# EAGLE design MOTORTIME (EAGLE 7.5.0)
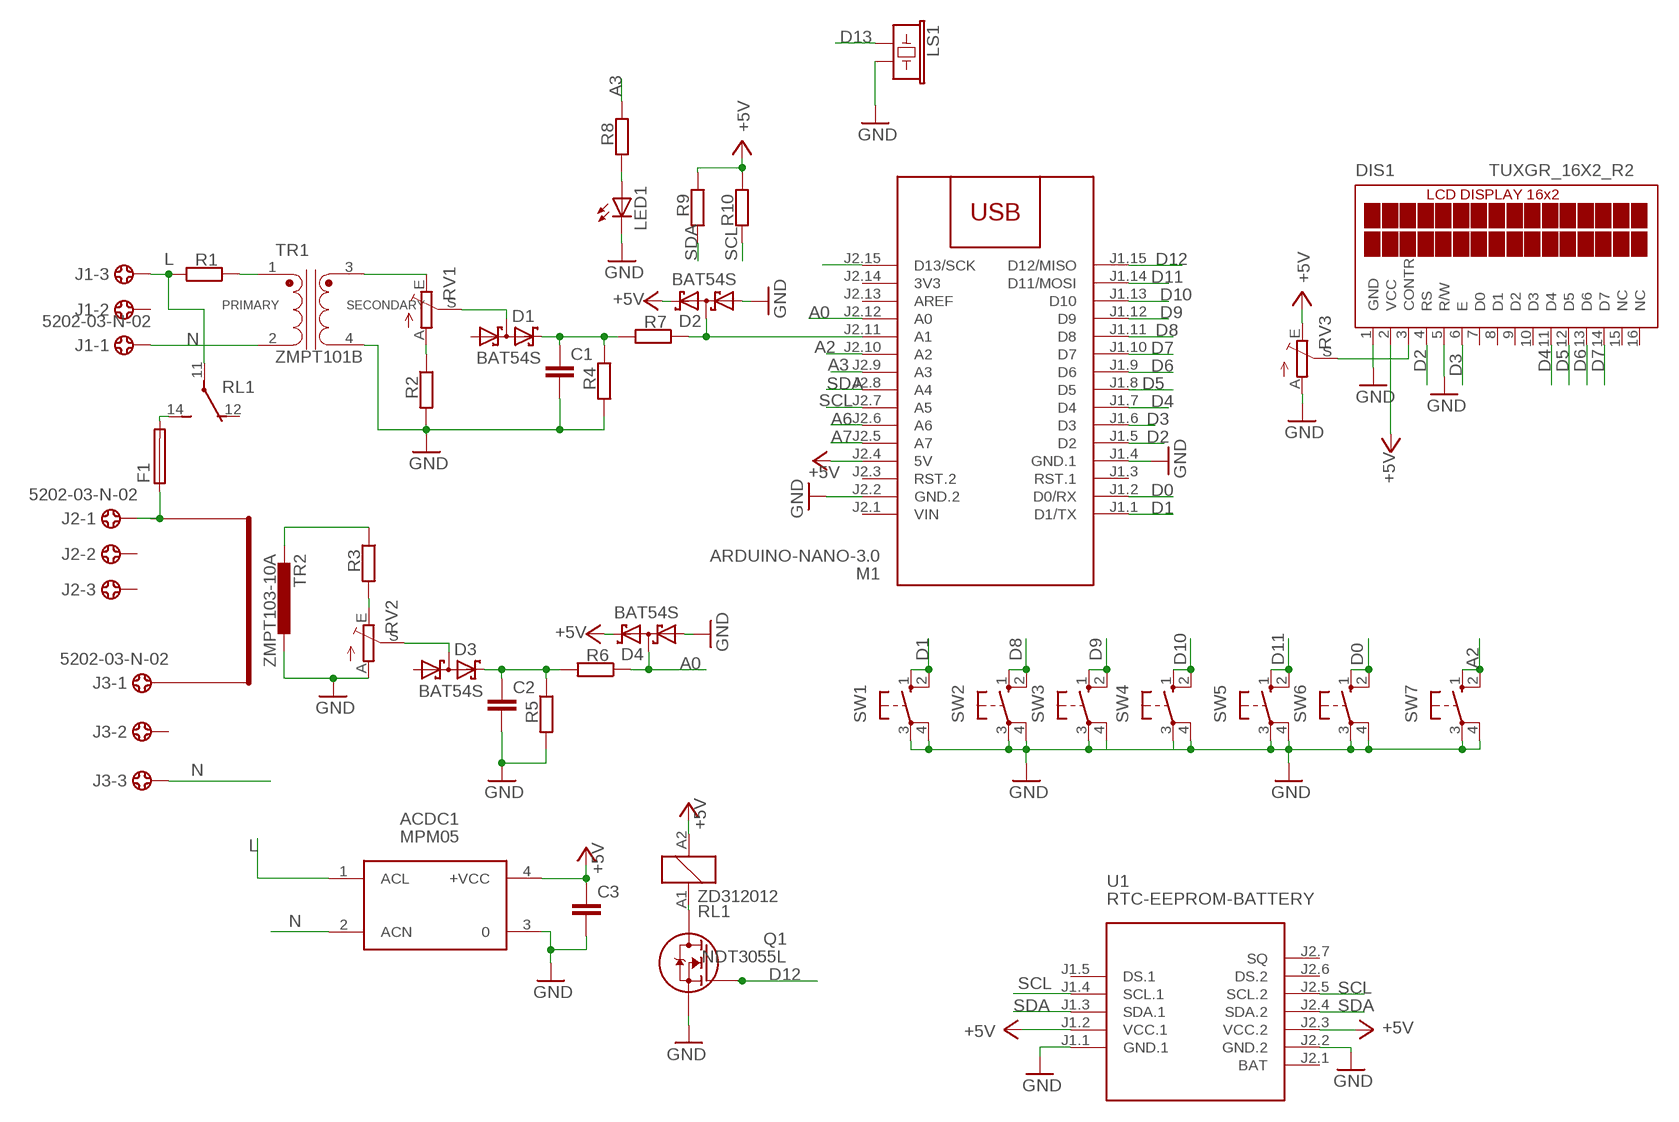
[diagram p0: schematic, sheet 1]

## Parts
ACDC1  MPM05  [MPM05]
C1  C-EUC1206  [C1206]
C2  C-EUC1206  [C1206]
C3  C-EUC1206  [C1206]
D1  BAT54S  [SOT23]
D2  BAT54S  [SOT23]
D3  BAT54S  [SOT23]
D4  BAT54S  [SOT23]
DIS1  TUXGR_16X2_R2  [TUXGR_16X2_R2]
F1  SH22,5A  [SH22,5A]
J1  5202-03-N-02  [5202-03-N-02]
J2  5202-03-N-02  [5202-03-N-02]
J3  5202-03-N-02  [5202-03-N-02]
LED1  LED5MM  [LED5MM]
LS1  BUZZER-PTH_NO_SILK  [BUZZER-12MM-NS]
M1  ARDUINO-NANO-3.0  [ARDUINO-NANO-3.0]
Q1  NDT3055L  [SOT223-4]
R1  R-EU_R1206  [R1206]
R2  R-EU_R1206  [R1206]
R3  R-EU_R1206  [R1206]
R4  R-EU_R1206  [R1206]
R5  R-EU_R1206  [R1206]
R6  R-EU_R1206  [R1206]
R7  R-EU_R1206  [R1206]
R8  R-EU_R1206  [R1206]
R9  R-EU_R1206  [R1206]
R10  R-EU_R1206  [R1206]
RL1  ZD312012  [ZD1]
RV1  TRIM_EU-B64W  [B64W]
RV2  TRIM_EU-B64W  [B64W]
RV3  TRIM_EU-B64W  [B64W]
SW1  10-XX  [B3F-10XX]
SW2  10-XX  [B3F-10XX]
SW3  10-XX  [B3F-10XX]
SW4  10-XX  [B3F-10XX]
SW5  10-XX  [B3F-10XX]
SW6  10-XX  [B3F-10XX]
SW7  10-XX  [B3F-10XX]
TR1  ZMPT101B  [XFMR_ZMPT101B]
TR2  ZMPT103-10A  [ZMPT103-10A]
U1  RTC-EEPROM-BATTERY  [RTC-EEPROM-BATTERY]

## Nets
+5V: ACDC1.4(+VCC) C3.1 D2.2(C2) D4.2(C2) DIS1.2(VCC) M1.J2.4(5V) R9.1 R10.1 RL1.A2 RV3.E U1.J1.2(VCC.1) U1.J2.3(VCC.2)
A0: D4.3(C1A2) M1.J2.12(A0) R6.1
A2: M1.J2.10(A2) SW7.1(S) SW7.2(S1)
A3: M1.J2.9(A3) R8.1
A6: M1.J2.6(A6)
A7: M1.J2.5(A7)
D0: M1.J1.2(D0/RX) SW6.1(S) SW6.2(S1)
D1: M1.J1.1(D1/TX) SW1.1(S) SW1.2(S1)
D2: DIS1.4(RS) M1.J1.5(D2)
D3: DIS1.6(E) M1.J1.6(D3)
D4: DIS1.11(D4) M1.J1.7(D4)
D5: DIS1.12(D5) M1.J1.8(D5)
D6: DIS1.13(D6) M1.J1.9(D6)
D7: DIS1.14(D7) M1.J1.10(D7)
D8: M1.J1.11(D8) SW2.1(S) SW2.2(S1)
D9: M1.J1.12(D9) SW3.1(S) SW3.2(S1)
D10: M1.J1.13(D10) SW4.1(S) SW4.2(S1)
D11: M1.J1.14(D11/MOSI) SW5.1(S) SW5.2(S1)
D12: M1.J1.15(D12/MISO) Q1.1(G)
D13: LS1.+ M1.J2.15(D13/SCK)
GND: ACDC1.3 C1.2 C2.2 C3.2 D2.1(A1) D4.1(A1) DIS1.1(GND) DIS1.5(R/W) LED1.K(C) LS1.- M1.J1.4(GND.1) M1.J2.2(GND.2) Q1.3(S) R2.2 R4.2 R5.2 RV2.A RV3.A SW1.3(P) SW1.4(P1) SW2.3(P) SW2.4(P1) SW3.3(P) SW3.4(P1) SW4.3(P) SW4.4(P1) SW5.3(P) SW5.4(P1) SW6.3(P) SW6.4(P1) SW7.3(P) SW7.4(P1) TR1.4 TR2.P$2 U1.J1.1(GND.1) U1.J2.2(GND.2)
L: ACDC1.1(ACL) J1.3 R1.2 RL1.11(2:P)
N: ACDC1.2(ACN) J1.1 J3.3 TR1.2
N$1: R2.1 RV1.A
N$2: R3.1 TR2.P$1
N$3: R3.2 RV2.E
N$4: F1.2 RL1.14(2:S)
N$5: R1.1 TR1.1
N$6: RV1.E TR1.3
N$7: C1.1 D1.2(C2) R4.1 R7.2
N$8: D1.3(C1A2) RV1.S
N$9: D2.3(C1A2) M1.J2.11(A1) R7.1
N$10: F1.1 J2.1
N$11: D3.3(C1A2) RV2.S
N$12: Q1.2(D) Q1.4(D) RL1.A1
N$13: C2.1 D3.2(C2) R5.1 R6.2
N$14: DIS1.3(CONTR) RV3.S
N$15: LED1.A R8.2
SCL: M1.J2.7(A5) R10.2 U1.J1.4(SCL.1) U1.J2.5(SCL.2)
SDA: M1.J2.8(A4) R9.2 U1.J1.3(SDA.1) U1.J2.4(SDA.2)
Unconnected: D1.1(A1) D3.1(A1) DIS1.7(D0) DIS1.8(D1) DIS1.9(D2) DIS1.10(D3) DIS1.15(NC) DIS1.16(NC) J1.2 J2.2 J2.3 J3.1 J3.2 M1.J1.3(RST.1) M1.J2.3(RST.2) M1.J2.13(AREF) RL1.12(2:O) U1.J1.5(DS.1) U1.J2.1(BAT) U1.J2.6(DS.2) U1.J2.7(SQ)

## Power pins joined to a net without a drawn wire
3V3: M1.J2.14(3V3)
VIN: M1.J2.1(VIN)

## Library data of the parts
ACDC1 = acdc:MPM05: AC DC Converter 5W
C1-C3 = rcl:C-EU: CAPACITOR, European symbol
D1-D4 = diode:BAT54S: Schottky Diodes Pin connection corrected 2011-05-04 Source: Fairchild .. BAT54.pdf
DIS1 = display-lcd:TUXGR_16X2_R2: Tuxgraphics LCD display 16x2 characters reflective, without background light Source: tuxgr_12x2_r2.pdf; OC_FARNELL: unknown; OC_NEWARK: unknown
F1 = fuse:SH22,5A: FUSE HOLDER; MPN: 0031.7701.11; OC_FARNELL: unknown; OC_NEWARK: 04F1224
J1-J3 = con-ebyelectro:5202-03-N-02: Barrier Blocks Sreies 5202 Source: http://www.ebyelectro.com/PDF/5202-XX-N-02.pdf; OC_FARNELL: unknown; OC_NEWARK: unknown
LED1 = led:LED: LED
LS1 = SparkFun-Electromechanical:BUZZER: Buzzer; PROD_ID: COMP-08253; SF_SKU: COM-07950
M1 = diy-modules:ARDUINO-NANO-3.0: Arduino Nano 3.0 and compatible devices More details available here: https://www.arduino.cc/en/Main/ArduinoBoardNano Click here to find device on ebay.com
Q1 = NDT3055L:NDT3055L: Trans MOSFET N-CH 60V 4A 4-Pin(3+Tab) SOT-223 Trans MOSFET N-CH 60V 4A 4-Pin(3+Tab) SOT-223 Check availability; AVAILABILITY: In Stock; CHECK_PRICES: https://www.snapeda.com/parts/NDT3055L/Onsemi/view-part/?ref=eda; DESCRIPTION: Trans MOSFET N-CH 60V 4A 4-Pin(3+Tab) SOT-223 Trans MOSFET N-CH 60V 4A 4-Pin(3+Tab) SOT-223; MF: ON; MP: NDT3055L; PACKAGE: SOT-223-4 Fairchild Semiconductor; PRICE: None; SNAPEDA_LINK: https://www.snapeda.com/parts/NDT3055L/Onsemi/view-part/?ref=snap
R1-R10 = rcl:R-EU_: RESISTOR, European symbol
RL1 = relay:ZD?1*: Power Relay SCHRACK 1 pole 30 A Source: http://www.schrack.com/.. 5848.pdf; OC_FARNELL: unknown; OC_NEWARK: unknown
RV1-RV3 = pot:TRIM_EU-: POTENTIOMETER
SW1-SW7 = switch-omron:10-XX: OMRON SWITCH; MPN: B3F-1000; OC_FARNELL: 176432; OC_NEWARK: 36M3542
TR1 = ZMPT101B:ZMPT101B: Check availability; AVAILABILITY: Not in stock; CHECK_PRICES: https://www.snapeda.com/parts/ZMPT101B/Qingxian+Zeming+Langxi+Electronic/view-part/?ref=eda; DESCRIPTION: Current-type Voltage Transformer; MF: Qingxian Zeming Langxi Electronic; MP: ZMPT101B; PACKAGE: None; PRICE: None; SNAPEDA_LINK: https://www.snapeda.com/parts/ZMPT101B/Qingxian+Zeming+Langxi+Electronic/view-part/?ref=snap
TR2 = diy-modules:ZMPT103-10A
U1 = diy-modules:RTC-EEPROM-BATTERY: RTC Module with Battery and EEPROM based on DS1307 and AT24C32 chips More details available here: http://henrysbench.capnfatz.com/henrys-bench/arduino-sensors-and-input/arduino-tiny-rtc-d1307-tutorial/ Click here to find device on ebay.com

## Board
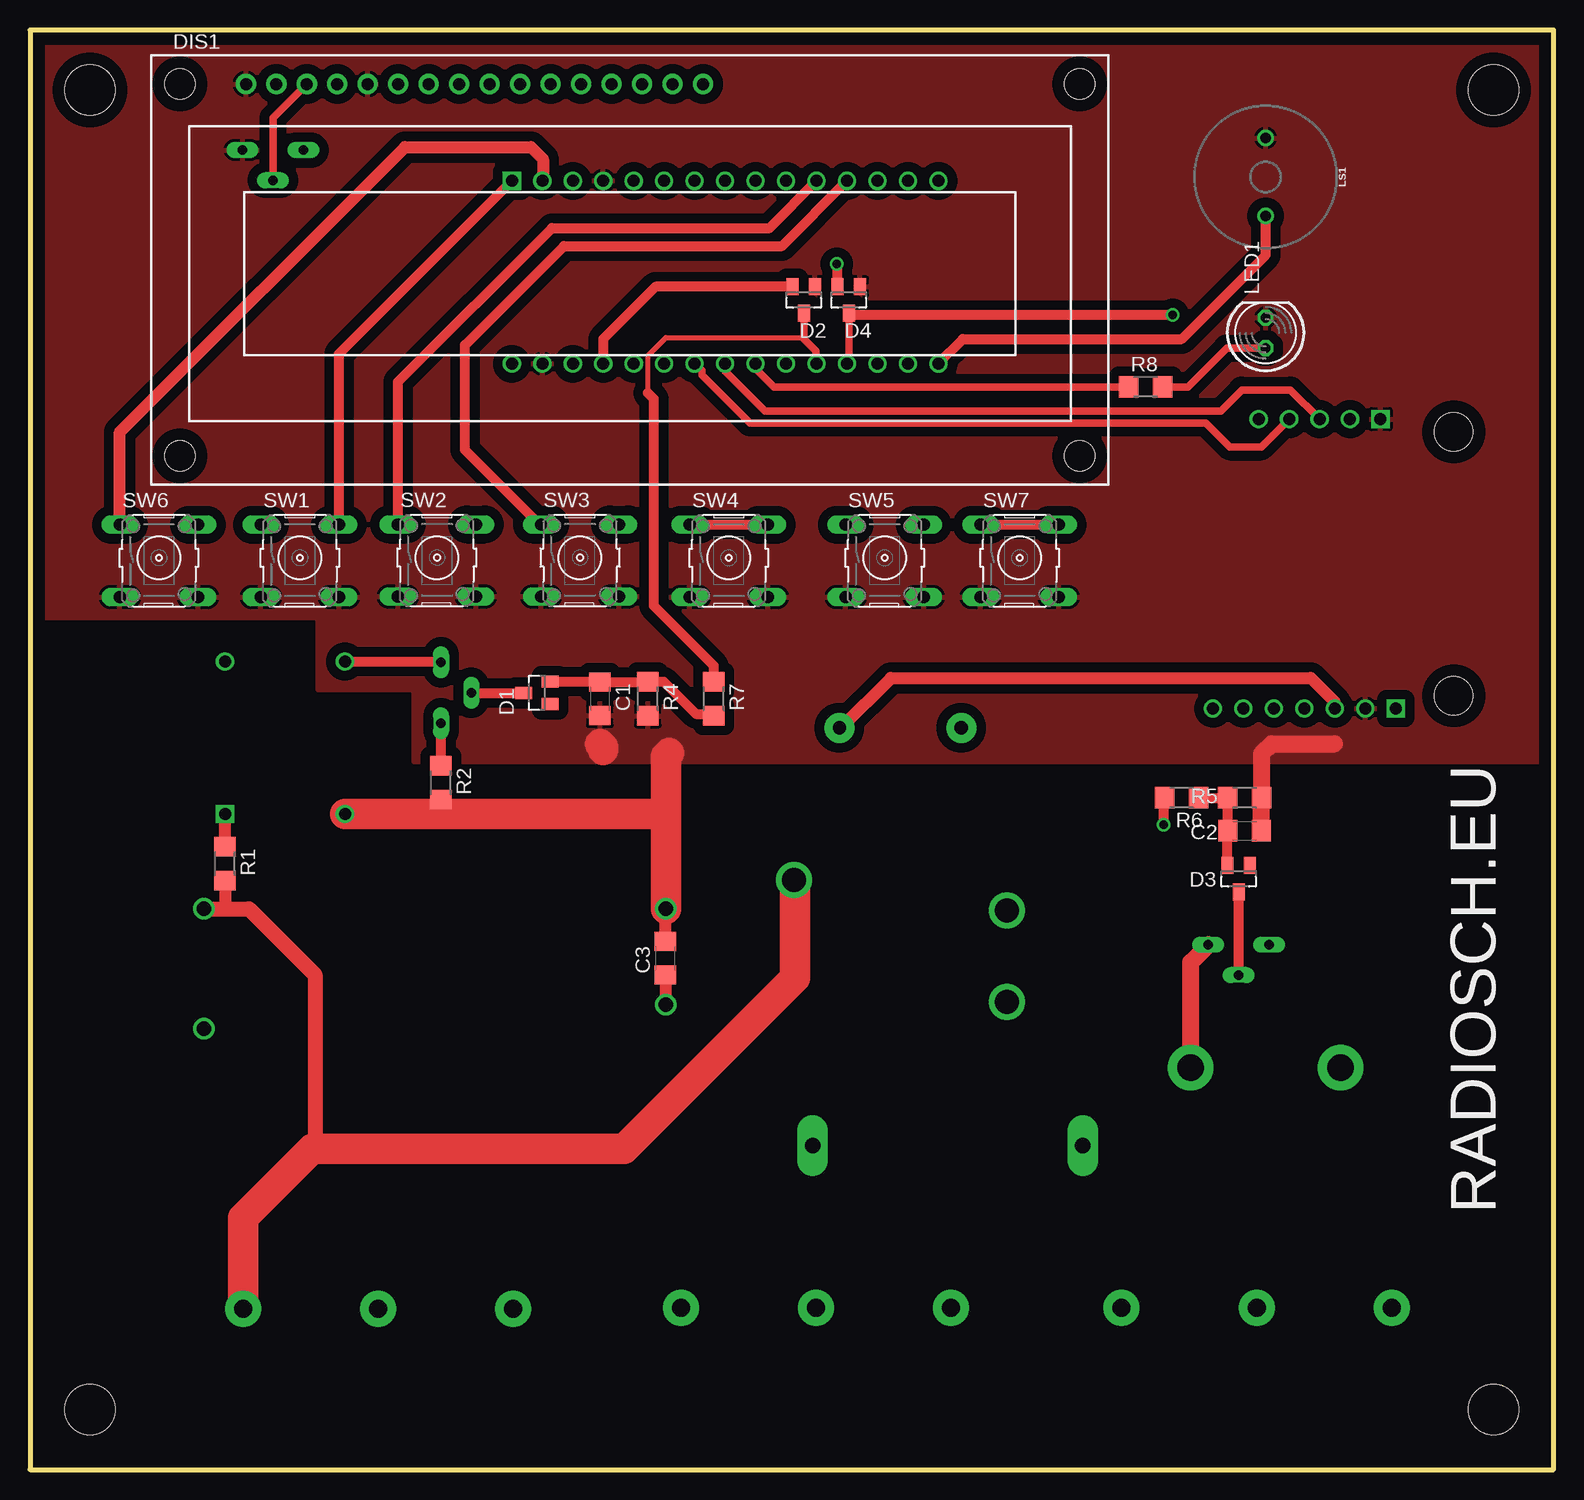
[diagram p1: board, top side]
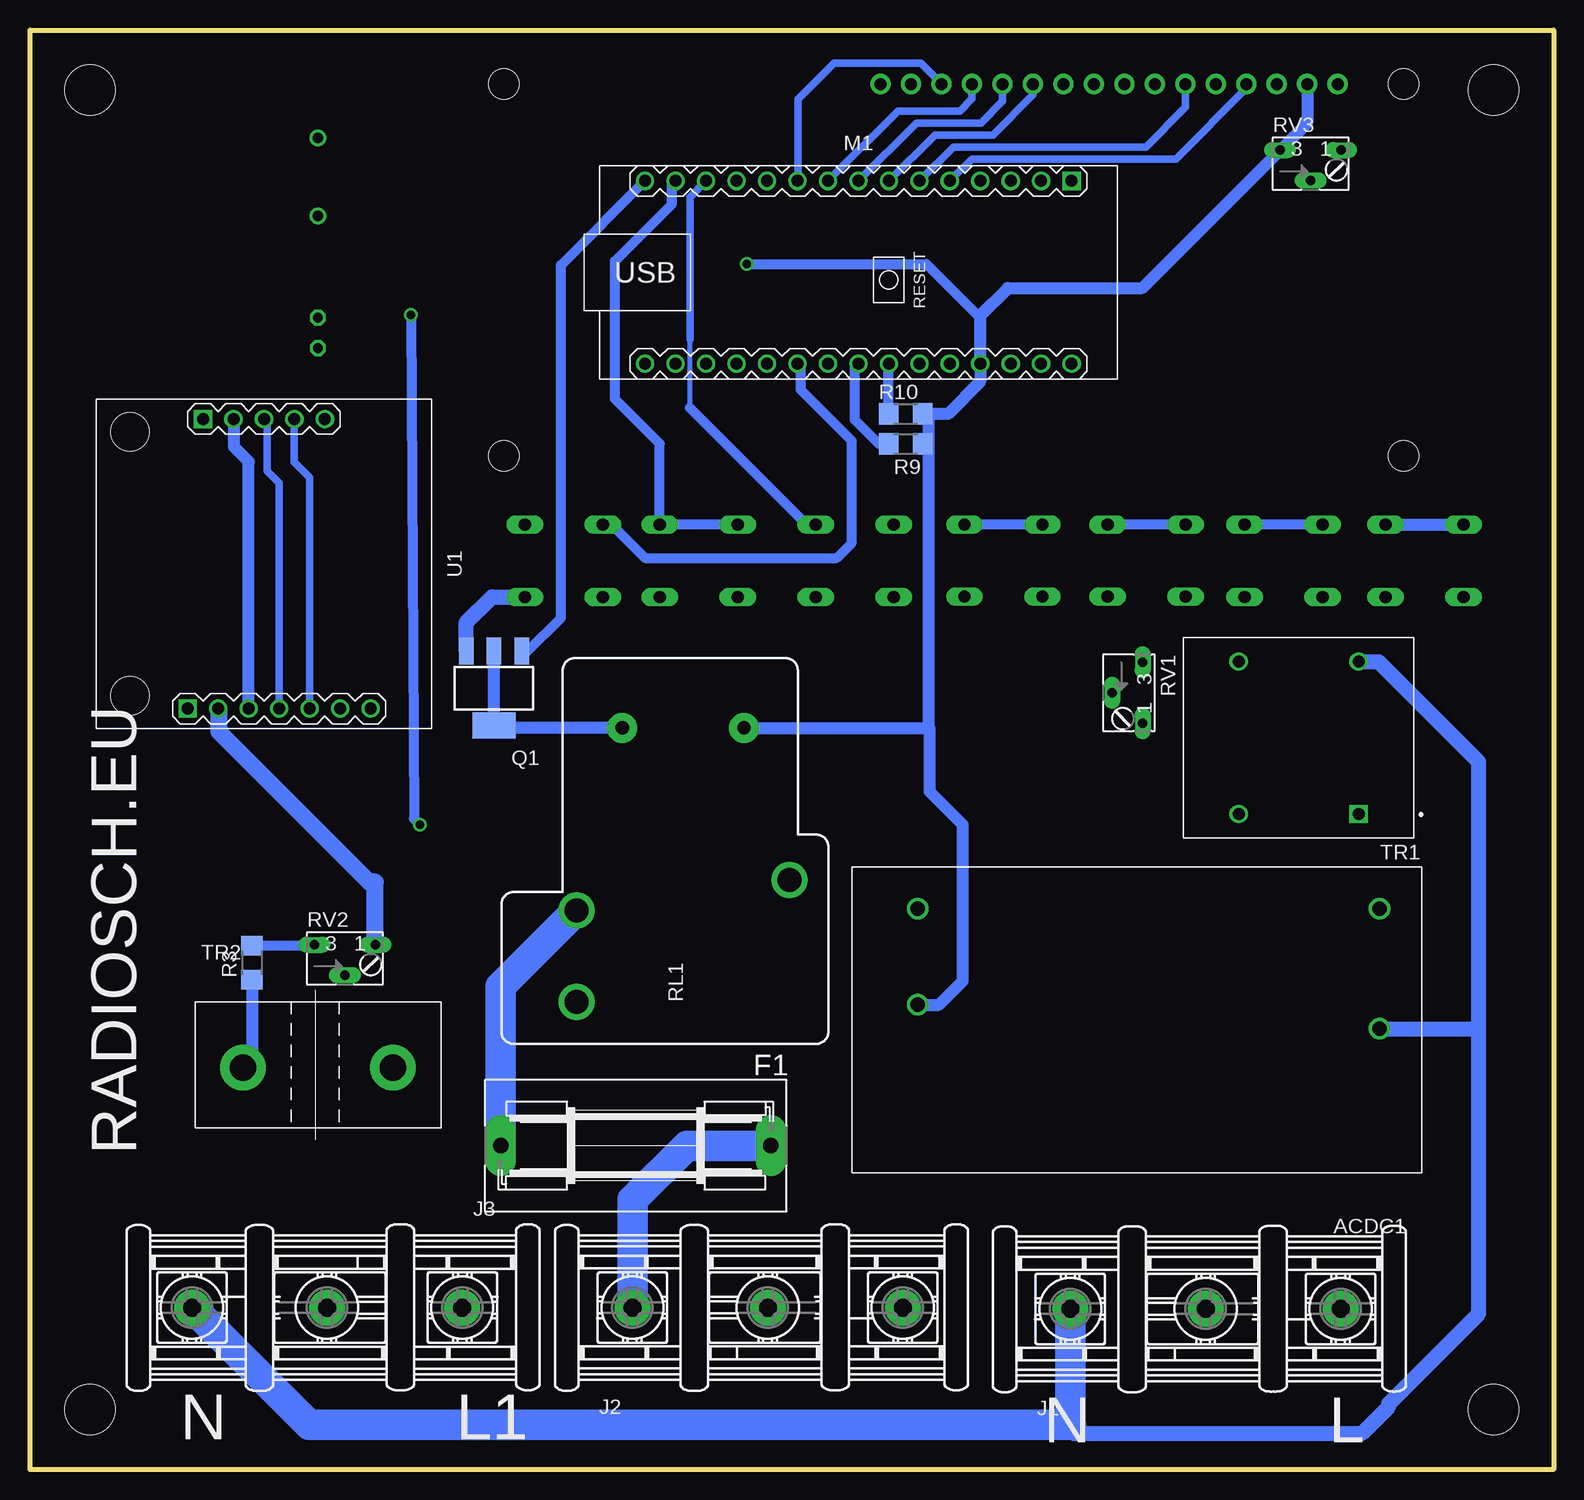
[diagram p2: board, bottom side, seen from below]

Size 127 x 120 mm. Coordinates in mm from the lower left corner, seen from the top.
Outline: 0,0 127,0 127,120 0,120 0,0
Copper layers (1*16): Top 0.035mm / dielectric 1.5mm / Bottom 0.035mm
Design rules "default": minimum track width 10mil, minimum drill 24mil, track to track 8mil, track to pad 8mil, pad to pad 8mil, via to via 8mil, smd to smd 8mil, copper to edge 40mil, drill to drill 8mil, minimum pad ring 10mil, minimum via ring 8mil, stop-mask expansion 4mil, vias tented up to drill 0mil, thermal gap 10mil
Holes 4.2 mm at 5,115 5,5 122,115 122,5

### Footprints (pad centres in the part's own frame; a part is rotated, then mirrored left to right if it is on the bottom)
MPM05 = drill 1.2: 1 3.5,-22; 2 3.5,-12; 3 42,-22; 4 42,-14
C1206 = smd 1.6 x 1.8: 1 -1.4,0; 2 1.4,0
SOT23 = smd 1 x 1.4: 1 -0.95,-1.1; 2 0.95,-1.1; 3 0,1.1
TUXGR_16X2_R2 = drill 1 pad 1.676: 1 -32,15.5; 2 -29.46,15.5; 3 -26.92,15.5; 4 -24.38,15.5; 5 -21.84,15.5; 6 -19.3,15.5; 7 -16.76,15.5; 8 -14.22,15.5; 9 -11.68,15.5; 10 -9.14,15.5; 11 -6.6,15.5; 12 -4.06,15.5; 13 -1.52,15.5; 14 1.02,15.5; 15 3.56,15.5; 16 6.1,15.5 | hole 2.5: -37.5,-15.5; 37.5,-15.5; -37.5,15.5; 37.5,15.5
SH22,5A = drill 1.321 pad 2.54 long: 1 -11.252,0; 2 11.252,0
5202-03-N-02 = drill 1.5 pad 3: 1 -9.29,0; 2 2,0; 3 13.25,0
LED5MM = drill 0.813 octagon: A -1.27,0; K 1.27,0
BUZZER-12MM-NS = drill 0.9: + 3.25,0; - -3.25,0
ARDUINO-NANO-3.0 = drill 1 square: J1.1 17.78,7.62 | drill 1: J1.2 15.24,7.62; J1.3 12.7,7.62; J1.4 10.16,7.62; J1.5 7.62,7.62; J1.6 5.08,7.62; J1.7 2.54,7.62; J1.8 0,7.62; J1.9 -2.54,7.62; J1.10 -5.08,7.62; J1.11 -7.62,7.62; J1.12 -10.16,7.62; J1.13 -12.7,7.62; J1.14 -15.24,7.62; J1.15 -17.78,7.62; J2.1 17.78,-7.62; J2.2 15.24,-7.62; J2.3 12.7,-7.62; J2.4 10.16,-7.62; J2.5 7.62,-7.62; J2.6 5.08,-7.62; J2.7 2.54,-7.62; J2.8 0,-7.62; J2.9 -2.54,-7.62; J2.10 -5.08,-7.62; J2.11 -7.62,-7.62; J2.12 -10.16,-7.62; J2.13 -12.7,-7.62; J2.14 -15.24,-7.62; J2.15 -17.78,-7.62
SOT223-4 = smd 1.219 x 2.235: 1 -2.24,-3.091; 2 0.071,-3.091; 3 2.383,-3.091 | smd 3.6 x 2.2: 4 0.071,3.107
R1206 = smd 1.6 x 1.803: 1 -1.422,0; 2 1.422,0
ZD1 = drill 2 pad 2.5: 11 -2.54,-8.88; 12 -12.7,8.88; 14 -5.08,8.88 | drill 1.1 pad 2.5: A1 10.16,5.08; A2 10.16,-5.08
B64W = drill 0.813 long: A 2.54,0; E -2.54,0; S 0,-2.54
B3F-10XX = drill 1.016 long: 1 -3.251,2.761; 2 3.251,2.761; 3 -3.251,-3.261; 4 3.251,-3.261
XFMR_ZMPT101B = drill 1 square: 1 -5,6.35 | drill 1: 2 -5,-6.35; 3 5,-6.35; 4 5,6.35
ZMPT103-10A = drill 2.2 pad 3.81: P$1 -1,-5; P$2 11.5,-5
RTC-EEPROM-BATTERY = drill 1 square: J1.1 -12.065,-5.08; J2.1 12.065,-6.35 | drill 1: J1.2 -12.065,-2.54; J1.3 -12.065,0; J1.4 -12.065,2.54; J1.5 -12.065,5.08; J2.2 12.065,-3.81; J2.3 12.065,-1.27; J2.4 12.065,1.27; J2.5 12.065,3.81; J2.6 12.065,6.35; J2.7 12.065,8.89 | hole 3.2: -11,-11.176; 11,-11.176

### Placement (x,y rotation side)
ACDC1  11,24.75 180 bottom
C1  47.5,64.25 270 top
C2  101.25,53.25 0 top
C3  52.97,42.62 90 top
D1  42.25,64.75 90 top
D2  64.5,97.5 180 top
D3  100.75,49.25 180 top
D4  68.25,97.5 180 top
DIS1  50,100 0 top
F1  76.5,27 180 bottom
J1  31,13.39 0 bottom
J2  67.5,13.5 0 bottom
J3  100.25,13.5 180 bottom
LED1  103,94.75 90 top
LS1  103,107.75 270 top
M1  57.95,99.8 0 bottom
Q1  88.25,65.12 180 bottom
R1  16.25,50.5 270 top
R2  34.25,57.25 270 top
R3  108.5,42.25 90 bottom
R4  51.5,64.25 270 top
R5  101.25,56 0 top
R6  96,56 0 top
R7  57,64.25 270 top
R8  93,90.25 0 top
R9  54,85.5 180 bottom
R10  54,88 180 bottom
RL1  72.55,51.67 90 bottom
RV1  34.25,64.75 270 bottom
RV2  100.75,43.75 0 bottom
RV3  20.25,110 0 bottom
SW1  22.5,76 0 top
SW2  33.92,76.02 0 top
SW3  45.85,76.02 0 top
SW4  58.25,76 0 top
SW5  71.25,76 0 top
SW6  10.75,76 0 top
SW7  82.5,76 0 top
TR1  21.25,61 180 bottom
TR2  108.25,38.5 0 bottom
U1  107.5,75.5 270 bottom

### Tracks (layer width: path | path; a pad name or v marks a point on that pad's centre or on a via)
+5V  (via drill 0.7)
  Top 0.813: D2.2 52.14,98.6 47.79,94.25 M1.J2.4 | D4.2 67.3,100.45 v67.25,100.5
  Top 1.016: RL1.A2 67.58,61.83 71.75,66 106.77,66 108.77,64 U1.J2.3 | C3.1 52.97,38.78 ACDC1.4
  Bottom 0.813: v67.25,100.5 52.29,100.5 47.79,96
  Bottom 1.016: ACDC1.4 51.25,38.75 49.25,40.75 49.25,53.75 52,56.5 52,61.75 52.08,61.83 | RL1.A2 52.08,61.83 | DIS1.2 20.54,112.25 RV3.E 34.29,98.5 45.5,98.5 47.79,96.21 47.79,96 M1.J2.4 47.79,90.71 50.5,88 R10.1 52.08,87.5 52.08,86 | U1.J2.3 108.77,84.02 110,85.25 110,87.53 U1.J1.2 | 52.08,61.83 52.08,86 | R9.1 52.08,86
A0  (via drill 0.7)
  Top 0.61: D4.3 68.25,92.32 M1.J2.12
  Top 0.813: v95.25,96.25 68.4,96.25 D4.3 | v94.5,53.75 94.5,55.92 R6.1
  Bottom 0.813: v95.25,96.25 95,54.25 v94.5,53.75
A2
  Top 0.813: SW7.1 SW7.2
  Bottom 0.813: SW7.1 78.51,78.76 75.75,76 59.75,76 58.5,77.25 58.5,85.75 62.75,90 62.75,91.9 M1.J2.10
A3
  Top 0.61: M1.J2.9 60.49,91.76 62,90.25 R8.1
D0
  Top 1.016: SW6.1 7.5,86.5 31.25,110.25 41.75,110.25 42.75,109.25 42.75,107.46 M1.J1.2
  Bottom 1.016: SW6.2 SW6.1
D1
  Top 0.813: SW1.2 25.75,93 M1.J1.1
  Bottom 0.813: SW1.1 SW1.2
D2
  Bottom 0.61: DIS1.4 25.62,115.13 31.5,109.25 48.5,109.25 M1.J1.5
D3
  Bottom 0.61: DIS1.6 30.7,113.55 34,110.25 50.04,110.25 M1.J1.6
D4
  Bottom 0.61: DIS1.11 43.4,114.6 46.75,111.25 51.58,111.25 M1.J1.7
D5
  Bottom 0.61: DIS1.12 45.94,114.06 47.75,112.25 53.12,112.25 M1.J1.8
D6
  Bottom 0.61: DIS1.13 48.48,114.27 49.5,113.25 54.66,113.25 M1.J1.9
D7
  Bottom 0.61: DIS1.14 51.02,115.52 52.75,117.25 60,117.25 63,114.25 63,107.45 M1.J1.10
D8
  Top 0.813: SW2.1 30.67,90.67 43.5,103.5 61.65,103.5 M1.J1.11
  Bottom 0.813: SW2.1 SW2.2
D9
  Top 0.813: SW3.1 42.47,78.78 36.25,85 36.25,93.75 44.5,102 62.69,102 M1.J1.12
  Bottom 0.813: SW3.1 SW3.2
D10
  Top 0.813: SW4.1 SW4.2
  Bottom 0.406: 72,88.5 72,94.25
  Bottom 0.61: 72,94.25 72,106.07 M1.J1.13
  Bottom 0.813: SW4.2 62.26,78.76 72,88.5
D11
  Bottom 0.813: M1.J1.14 73.5,107.11 73.5,105.5 78.25,100.75 78.25,89.25 74.5,85.5 SW5.2 SW5.1
D12
  Bottom 0.813: Q1.1 85.53,68.22 82.75,71 82.75,100.4 M1.J1.15
D13
  Top 0.813: M1.J2.15 75.73,92.23 77.75,94.25 96,94.25 103,101.25 LS1.+
GND
  Top 1.016: R2.2 34.25,55.15 34.75,54.65 | C3.2 52.97,46.72 ACDC1.3
  Top 1.422: 108.75,60.5 103.5,60.5 102.67,59.67 R5.2 102.65,55.98 C2.2 | TR2.P$2 96.75,42.29 RV2.A
  Top 2.54: TR1.4 34.75,54.65 52.6,54.65 53,54.25 | 47.75,60 47.75,60.25 47.5,60.5 | ACDC1.3 53,54.25 | 53,54.25 53,59.5 53.25,59.75
  Bottom 1.27: Q1.3 90.63,70.62 88.5,72.75 85.76,72.75 SW7.4
  Bottom 1.422: RV2.A 98.21,48.96 98.71,48.96 111.25,61.5 111.25,63.38 U1.J2.2
  pour Top (isolate 0.813): 0,119 126,119 126,59 32,59 32,65 24,65 24,71 0,71
L
  Top 1.016: R1.2 16.25,46.75
  Top 1.27: ACDC1.1 16.25,46.75 18.25,46.75 23.75,41.25 23.75,27 24,26.75
  Top 2.54: J1.3 17.75,21 23.5,26.75 24,26.75 49.5,26.75 63.75,41 63.75,49.05 RL1.11
N
  Bottom 1.27: TR1.2 14.6,67.35 6.25,59 6.25,36.75 | J1.1 40.29,5.54 40.25,5.5 | 6.25,36.75 6.25,13 13.75,5.5 13.75,5.25 16,3 40,3 40.75,3.75 | ACDC1.2 6.25,36.75
  Bottom 2.54: J1.1 40.29,3.79 40.25,3.75 40.75,3.75 103.75,3.75 J3.3
N$1
  Top 0.813: R2.1 RV1.A
N$2
  Bottom 1.016: R3.1 108.5,34.25 TR2.P$1
N$3
  Bottom 0.813: R3.2 103.37,43.67 RV2.E
N$4
  Bottom 2.54: F1.2 87.75,40.27 RL1.14
N$5
  Top 1.016: R1.1 TR1.1
  Top 1.27: 16.23,54.67 TR1.1
N$6
  Top 0.813: TR1.3 34.19,67.35 RV1.E
N$7
  Top 0.813: D1.2 47.45,65.7 C1.1 51.48,65.65 R4.1 52.83,65.67 55.5,63 56.83,63 R7.2
N$8
  Top 0.813: RV1.S D1.3
N$9
  Top 0.406: 51.5,89.75 51.5,92.88 53,94.38 64.38,94.38 64.5,94.5
  Top 0.61: D2.3 64.5,94.5 64.5,94.25 65.5,93.25 65.5,92.25 M1.J2.11
  Top 0.813: 51.5,89.75 52,89.25 52,72 57,67 R7.1
N$10
  Bottom 2.54: J2.1 76.79,22.46 72.25,27 F1.1
N$11
  Top 0.813: RV2.S D3.3
N$12
  Bottom 1.016: RL1.A1 88.13,61.83 Q1.4 Q1.2
N$13
  Top 0.813: D3.2 99.8,53.2 C2.1 99.85,55.98 R5.1 R6.2
N$14
  Top 0.61: RV3.S 20.25,112.67 DIS1.3
N$15
  Top 0.61: R8.2 96.5,90.25 99.75,93.5 102.98,93.5 LED1.A
SCL
  Top 0.61: 104.96,87.79 U1.J1.4 102.64,85.25 100,85.25 98,87.25 60,87.25 56,91.25 56,91.59 M1.J2.7
  Bottom 0.61: U1.J2.5 103.69,82.69 105,84 105,87.53 U1.J1.4
  Bottom 0.813: R10.2 55.42,92.17 M1.J2.7
SDA
  Top 0.61: M1.J2.8 57.95,91.55 61.25,88.25 99.25,88.25 101,90 105.06,90 U1.J1.3
  Bottom 0.61: U1.J2.4 106.23,82.23 107.25,83.25 107.25,87.31 U1.J1.3
  Bottom 0.813: R9.2 56.25,85.5 58.25,87.5 58.25,91.88 M1.J2.8

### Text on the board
tPlace: RADIOSCH.EU
bPlace: RADIOSCH.EU | L | N | L1 | N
